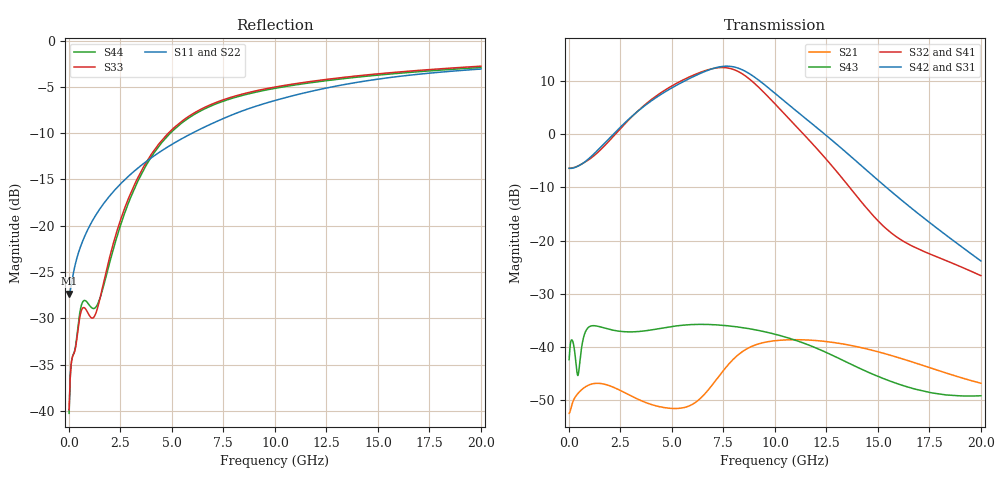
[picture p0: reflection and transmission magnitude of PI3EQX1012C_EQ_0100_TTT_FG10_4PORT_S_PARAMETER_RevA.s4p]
! NPort=4 DATA=2000 NOISE=0 GROUPDELAY=0 COMPLEX_DATAFORMAT=POLAR
! NumOfBlock=1 NumOfParam=0
! .MODEL Smodel S TSTONEFILE=PI3EQX1012C_EQ_0100_TTT_FG10_4PORT_S_PARAMETER_RevA.s4p TYPE=S
!  -- The above .MODEL line can be used for the S element in the netlist.
! The s parameter is extracted from the linear redriver, it is not bi-directional; only s(4,1)s(4,2) and s(3,1)s(3,2)
! should be the insertion loss
!Port definition:
!Port1 = input+
!Port2 = input-
!Port3 = output+
!Port4 = output-
# Hz S MA R  50
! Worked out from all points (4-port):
!   2000 points, 10 MHz to 20 GHz, reference 50 ohm
!   strongest paths, dB at 10 MHz, 5.01 GHz, 10.01 GHz, 15.01 GHz, 20 GHz:
!     S42: -6.4, 8.7, 7.7, -8.7, -23.8
!     S31: -6.4, 8.7, 7.6, -8.9, -24.2
!     S32: -6.4, 9.1, 5.7, -16.3, -26.6
!     S41: -6.4, 9.1, 5.8, -16.5, -26.9
!     S43: -42.4, -36.1, -37.6, -45.5, -49.1
!     S21: -52.4, -51.5, -38.8, -40.9, -46.8
!   lowest |S11| = -27.3 dB at 10 MHz (marker M1), VSWR 1.09, Z = 45.9 - j0.123 ohm
!   |S11| at or under -10 dB: start of sweep to 5.988 GHz
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1e7  0.04301 -178.2  0.002379 1.5  0.0008102 -0.5  0.0008039 -0.5
     0.002388 1.5  0.04109 -178.1  0.000927 -0.5  0.0009197 -0.5
     0.4784 -0.2  0.4775 179.9  0.01016 -4.0  0.007598 -25.7
     0.4771 179.9  0.4794 -0.2  0.007615 -25.8  0.009722 -4.0
4.12e9  0.2379 -124.3  0.00288 0.2  0.0003795 -57.0  0.0003778 -57.3
        0.002843 0.4  0.2415 -123.2  0.0004313 -57.6  0.0004293 -58.0
        2.135 -65.5  2.199 126.3  0.2544 -83.8  0.01363 33.4
        2.187 127.0  2.134 -63.8  0.01462 30.5  0.2464 -83.5
5.8e9  0.3085 -123.9  0.002837 32.4  0.0002752 -58.3  0.000274 -59.3
       0.002782 31.2  0.3136 -123.2  0.0003119 -59.3  0.0003107 -60.2
       3.279 -131.6  3.416 59.7  0.3887 -99.9  0.01642 8.6
       3.427 60.0  3.294 -129.7  0.01621 6.0  0.3809 -99.7
7.13e9  0.3639 -124.6  0.005086 53.3  0.0002377 -55.8  0.0002356 -57.1
        0.004873 53.6  0.3694 -124.1  0.000268 -57.0  0.0002657 -58.3
        4.184 165.4  4.183 -3.9  0.4626 -110.1  0.01666 -11.9
        4.216 -4.1  4.211 167.5  0.01619 -13.1  0.4544 -109.9
8.28e9  0.4115 -126.0  0.008896 40.4  0.0002224 -54.1  0.0002193 -55.6
        0.008655 41.6  0.4176 -125.5  0.0002491 -55.4  0.0002457 -56.9
        4.103 101.0  3.824 -68.2  0.5092 -116.8  0.01574 -27.5
        3.868 -68.7  4.132 103.4  0.01538 -28.0  0.5007 -116.7
9.63e9  0.4617 -128.2  0.01136 14.3  0.000213 -53.9  0.0002089 -55.5
        0.01121 15.5  0.4686 -127.8  0.000237 -55.1  0.0002326 -56.6
        2.756 32.6  2.293 -134.8  0.551 -122.8  0.01407 -43.5
        2.326 -135.9  2.779 35.3  0.01377 -44.1  0.5422 -122.7
2e10  0.7017 -144.6  0.004644 -67.3  0.0001465 -72.3  0.0001414 -73.8
      0.004578 -66.6  0.7167 -144.3  0.0001625 -72.1  0.0001568 -73.7
      0.06135 107.5  0.04688 34.8  0.7272 -143.5  0.00357 -51.6
      0.04527 33.1  0.06446 112.3  0.003489 -48.9  0.7152 -143.3
